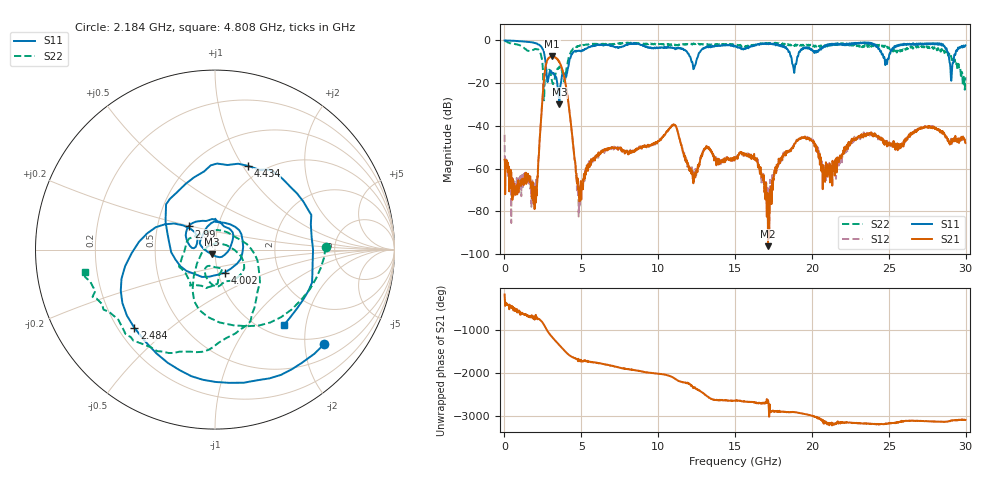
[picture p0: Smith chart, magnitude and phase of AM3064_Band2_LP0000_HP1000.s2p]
# Hz S DB R 50.0
!freq dBS11 angS11 dBS21 angS21 dBS12 angS12 dBS22 angS22
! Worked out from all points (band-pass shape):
!   1600 points, 10 MHz to 29.98 GHz, reference 50 ohm
!   highest |S21| = -7.53 dB at 3.103 GHz (marker M1); lowest = -96.3 dB at 17.14 GHz (marker M2)
!   |S21| within 3 dB of the highest: 2.729 GHz to 3.596 GHz (867.3 MHz wide, 27.4 % of centre)
!   lowest |S11| = -29.9 dB at 3.571 GHz (marker M3), VSWR 1.07, Z = 48.3 - j2.63 ohm
!   |S11| at or under -10 dB: 2.67 GHz to 4.208 GHz (1.538 GHz wide, 44.7 % of centre); 12.17 GHz to 12.47 GHz (301.9 MHz wide, 2.45 % of centre); 18.7 GHz to 19 GHz (296.4 MHz wide, 1.57 % of centre)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
!   |S22| runs from -28.0 to -0.2 dB; largest |S21 - S12| = 0.0096
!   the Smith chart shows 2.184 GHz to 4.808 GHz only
!   S11 on the Smith chart (normalised r, x): 2.184 GHz: 0.82, -2.44; 2.484 GHz: 0.27, -0.38; 2.99 GHz: 0.72, +0.19; 4.002 GHz: 1.08, -0.28; 4.434 GHz: 0.84, +1.05; 4.808 GHz: 1.21, -1.51
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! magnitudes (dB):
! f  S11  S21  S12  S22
! 10 MHz  0.0  -55.8  -44.2  -0.2
! 591.1 MHz  -0.2  -70.4  -69.1  -1.6
! 1.941 GHz  -1.2  -71.2  -72.9  -4.2
! 2.184 GHz  -1.9  -60.0  -60.2  -4.2
! 2.484 GHz  -4.1  -25.7  -25.7  -11.8
! 2.99 GHz  -14.2  -7.8  -7.8  -14.9
! 3.103 GHz  -15.6  -7.5  -7.6  -19.5
! 3.571 GHz  -29.9  -10.1  -10.0  -12.2
! 4.002 GHz  -17.1  -21.4  -21.4  -14.9
! 4.434 GHz  -6.0  -46.2  -46.3  -4.1
! 4.808 GHz  -4.9  -68.8  -74.4  -2.7
! 5.015 GHz  -5.0  -68.0  -68.7  -2.5
! 10 GHz  -3.4  -47.2  -47.1  -1.7
! 11.09 GHz  -3.9  -39.7  -39.5  -1.9
! 12.31 GHz  -13.4  -65.2  -64.2  -1.7
! 15 GHz  -2.6  -55.1  -54.5  -1.9
! 16.32 GHz  -2.1  -55.4  -55.9  -1.9
! 17.14 GHz  -1.6  -96.3  -73.4  -1.3
! 19.99 GHz  -4.4  -47.0  -46.9  -2.2
! 20.85 GHz  -2.8  -66.2  -61.4  -2.8
! 25 GHz  -8.4  -48.6  -48.3  -3.2
! 29.98 GHz  -2.3  -48.0  -46.4  -17.3
